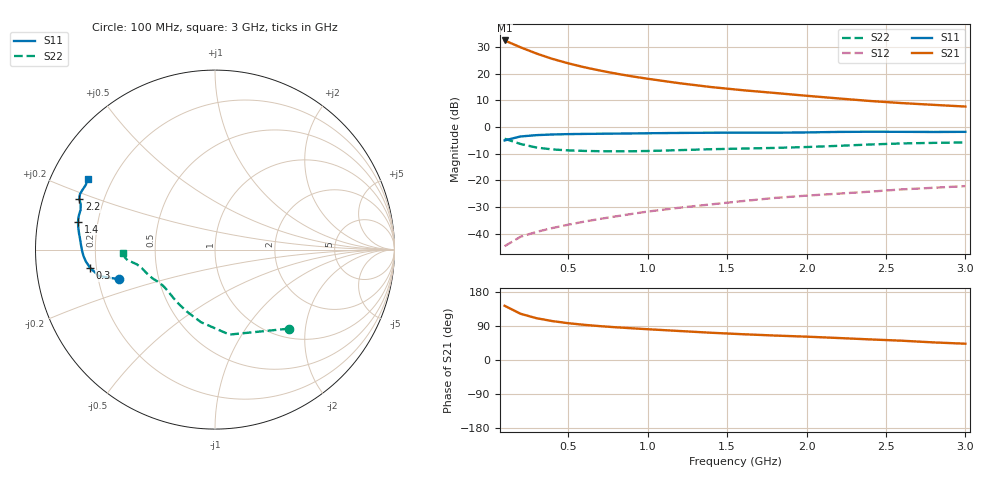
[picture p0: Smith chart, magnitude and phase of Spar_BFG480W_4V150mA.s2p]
! Filename: 4150BFG480.001
! Title: BFG480W
! Bias: Vce=4V; Ic=150mA
! Company: NXP Semiconductors NL
! User: Quality&Reliability T&D
! Measure time: 10 Nov 1999 / 12:05:01
#  MHz  S  MA  R 50
! Freq  S11  S21  S12  S22  :
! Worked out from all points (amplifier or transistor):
!   20 points, 100 MHz to 3 GHz, reference 50 ohm
!   highest |S21| = 32.4 dB at 100 MHz (marker M1)
!   |S21| within 3 dB of that: start of sweep to 219.1 MHz
!   unconditionally stable (mu >= 1): 414.3 MHz to end of sweep
!   at 400 MHz: K = 0.99, MSG = 31.7 dB, |S12| = -37.9 dB
!   at 1.2 GHz: K = 1.16, MAG = 20.9 dB, |S12| = -30.3 dB
!   at 3 GHz: K = 1.10, MAG = 12.9 dB, |S12| = -22.1 dB
!   S11 on the Smith chart (normalised r, x): 100 MHz: 0.29, -0.14; 300 MHz: 0.18, -0.07; 1.4 GHz: 0.13, +0.10; 2.2 GHz: 0.11, +0.18; 3 GHz: 0.11, +0.26
100  0.5597 -162.8  41.66 143.1  0.005854 65.0  0.6024 -47.0
200  0.6631 -167.2  31.04 122.0  0.008791 59.3  0.4804 -80.3
300  0.7026 -171.6  23.75 110.4  0.01081 60.0  0.4119 -100.9
400  0.7229 -174.8  18.85 102.7  0.01278 62.9  0.3796 -114.3
500  0.7339 -177.3  15.57 97.2  0.01476 65.8  0.364 -123.6
600  0.7408 -179.5  13.16 92.9  0.01684 67.9  0.3558 -130.2
700  0.7457 178.5  11.39 89.4  0.01896 70.2  0.3513 -135.3
800  0.7506 176.7  9.996 86.3  0.02114 71.8  0.3497 -139.4
900  0.7557 175.0  8.882 83.7  0.02351 73.5  0.3508 -143.0
1000  0.7619 173.5  7.994 81.2  0.02602 74.5  0.3545 -146.3
1200  0.7723 170.7  6.595 76.5  0.03071 75.9  0.3679 -151.5
1400  0.7791 168.4  5.584 71.9  0.03551 76.7  0.3829 -155.2
1600  0.782 166.1  4.872 68.0  0.04095 77.2  0.3937 -158.3
1800  0.7808 163.6  4.331 64.6  0.04684 77.6  0.4051 -161.7
2000  0.7893 161.5  3.836 61.6  0.05175 78.0  0.4208 -165.8
2200  0.8071 159.4  3.422 58.1  0.05638 77.8  0.443 -169.3
2400  0.8136 157.6  3.064 54.3  0.06141 77.1  0.4694 -171.6
2600  0.8101 155.9  2.797 50.9  0.06773 76.4  0.4911 -173.1
2800  0.8053 153.5  2.594 46.4  0.0726 74.8  0.5032 -174.9
3000  0.8098 150.8  2.409 43.0  0.07808 73.9  0.513 -177.7
